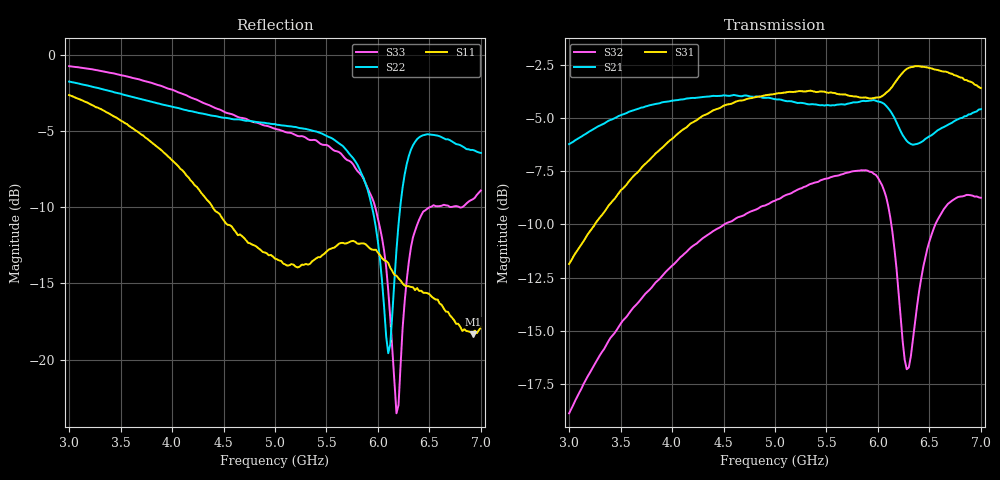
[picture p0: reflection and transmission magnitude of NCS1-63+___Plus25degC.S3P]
! Mini-Circuits
! S3P DATA File Format
! Type: Transmission Line Balun
! Model: NCS1-63+
! TEST CONDITIONS: INPUT POWER = 0 dBm @ Temperature = +25deg C
! TB-419+ using open port de-emebeding to temrinal edge
! 401 Frequency points
! All S Parameters are in dB deg format
! Port 1 is input port 2 & 3 are outputs
! Tested using E5071C with Port Z conversion for Port 2 & 3 set to 25 Ohm
# Hz S dB R 50
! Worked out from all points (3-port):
!   201 points, 3 GHz to 7 GHz, reference 50 ohm
!   strongest paths, dB at 3 GHz, 4 GHz, 5 GHz, 6 GHz, 7 GHz:
!     S31: -11.9, -6.0, -3.9, -4.0, -3.6
!     S21: -6.2, -4.2, -4.1, -4.2, -4.6
!     S32: -18.9, -11.9, -8.9, -7.8, -8.7
!   lowest |S11| = -18.3 dB at 6.92 GHz (marker M1), VSWR 1.28, Z = 41.3 + j6.87 ohm
!   |S11| at or under -10 dB: 4.394 GHz to end of sweep
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3e9  -2.65 118.0  -6.33 -27.7  -12.01 144.6
     -6.23 -27.8  -1.77 10.2  -18.85 54.8
     -11.85 144.0  -18.86 55.1  -0.76 3.6
3.94e9  -6.53 30.5  -4.28 -88.3  -6.33 82.3
        -4.25 -88.1  -3.32 -16.4  -12.31 3.5
        -6.23 82.1  -12.22 4.7  -2.17 -28.0
5e9  -13.37 -109.2  -4.05 -156.9  -3.82 15.1
     -4.13 -156.4  -4.56 -42.2  -8.95 -61.1
     -3.88 15.6  -8.89 -60.9  -4.86 -55.5
5.94e9  -12.78 146.7  -4.08 143.9  -4.02 -31.9
        -4.18 143.3  -9.93 -123.4  -7.37 -154.3
        -4.09 -30.2  -7.54 -156.1  -9.34 -120.4
6.1e9  -13.66 135.6  -4.48 130.1  -3.66 -36.0
       -4.55 129.8  -19.57 132.4  -9.24 157.3
       -3.75 -35.0  -9.14 155.3  -15.45 -170.4
6.18e9  -14.49 132.4  -5.19 124.2  -3.19 -39.2
        -5.20 124.0  -12.80 34.8  -12.34 114.1
        -3.25 -38.8  -12.04 113.5  -23.51 102.4
6.3e9  -15.18 130.5  -6.27 122.8  -2.65 -47.4
       -6.17 121.9  -6.65 -25.4  -16.41 -0.3
       -2.65 -48.2  -16.70 1.7  -13.59 -26.6
6.48e9  -15.63 124.2  -5.96 121.3  -2.65 -60.8
        -5.93 120.0  -5.22 -79.7  -11.14 -95.9
        -2.64 -62.2  -11.13 -96.1  -10.10 -84.1
6.92e9  -18.31 137.6  -4.80 98.8  -3.37 -89.4
        -4.76 96.9  -6.25 -164.6  -8.33 -179.8
        -3.35 -89.1  -8.65 -179.3  -9.49 174.4
7e9  -17.87 144.6  -4.61 94.1  -3.58 -94.9
     -4.60 92.2  -6.44 -177.2  -8.35 168.3
     -3.60 -94.4  -8.75 168.0  -8.91 157.4
